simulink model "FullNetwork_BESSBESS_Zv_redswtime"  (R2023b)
settings: Solver=ode15s  StartTime=0.0  StopTime=140  RelTol=1e-3
PreLoadFcn:
  | Ts=50e-6;
model workspace (MAT data in the model file):
  Cf1 = 0.02
  Cf2 = 0.02
  Kffi1 = 0.9
  Kffi2 = 0.9
  Kffi3 = 0.9
  Kffv1 = 1
  Kffv2 = 1
  Kffv3 = 1
  Ki_cc1 = 5.9
  Ki_cc2 = 5.9
  Ki_cc3 = 5.9
  Ki_q1 = 0.0001
  Ki_q2 = 0.0001
  Ki_q3 = 0.0001
  Ki_vc1 = 150
  Ki_vc2 = 150
  Ki_vc3 = 150
  Kp_cc1 = 0.015
  Kp_cc2 = 0.015
  Kp_vc1 = 5
  Kp_vc2 = 5
  Kp_vc3 = 5
  Lf1 = 4.75e-06
  Lf2 = 4.75e-06
  Rf1 = 0.0005
  Rf2 = 0.0005
  Rf3 = 0.0005
  Rv1 = 0.0003169
  Rv2 = 0.0003169
  Snom1 = 100000000
  Snom2 = 100000000
  Vdc1 = 2000
  Vdc2 = 2000
  Vdc3 = 2000
  Xv1 = 0.0009509
  Xv2 = 0.0009509
  fnom1 = 50
  fnom2 = 50
  mp1 = 6.25e-08
  mp2 = 6.25e-08
  nq1 = 4.69166666667e-07
  nq2 = 4.69166666667e-07
  tau1 = 0.001
  tau2 = 0.001
  tau3 = 0.001
  vnom1 = 690
  vnom2 = 690
  vnom3 = 690
undefined symbols (not defined in the file or in its folder): Armidale, DiscIntNeverNeededParam, find_system, Gunnedah, Innerell, Ion, Lithium, Morree, Narrabri, Tamworth
libraries: spsThreePhaseBreakerLib x41, spsThreePhaseVIMeasurementLib x16, simulink_extras x16, spsThreePhaseSeriesRLCLoadLib x14, spsabctodq0Lib x12, spsThreePhaseTransformerTwoWindingsLib x11, slpidlib x8, spsLoadFlowBusLib x8, spsThreePhasePISectionLineLib x8, powerlib_extras x7, spsFirstOrderFilterLib x6, simulink x5
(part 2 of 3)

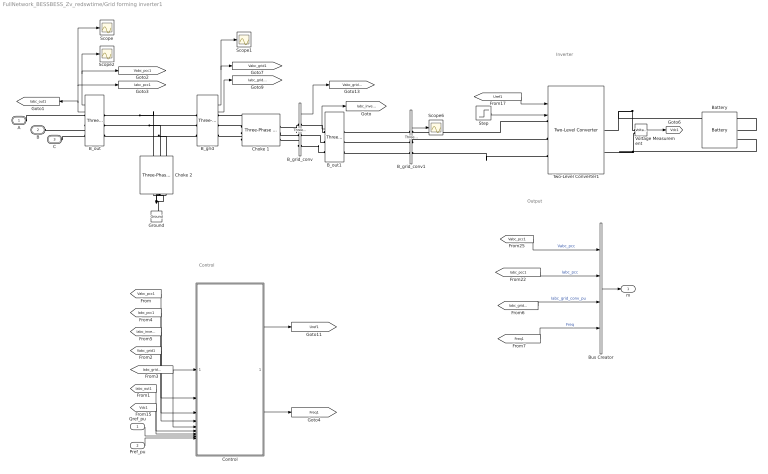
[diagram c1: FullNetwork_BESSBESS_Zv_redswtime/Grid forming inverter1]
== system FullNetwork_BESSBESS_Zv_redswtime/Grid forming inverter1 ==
  note: Control
  note: Inverter
  note: Output
  Qref_pu : Inport
  Pref_pu : Inport  Port=2
  B_grid : spsThreePhaseVIMeasurementLib/Three-Phase V-I Measurement  VoltageMeasurement=phase-to-ground  SetLabelV=off  LabelV=Vabc  Vpu=on  VpuLL=off  CurrentMeasurement=yes  SetLabelI=off  LabelI=Iabc  Ipu=on  Pbase=100e6  Vbase=690  OutputType=Complex  PhasorSimulation=off  PSBequivalent=0
  B_grid_conv : spsThreePhaseVIMeasurementLib/Three-Phase V-I Measurement  VoltageMeasurement=phase-to-ground  SetLabelV=off  LabelV=Vabc  Vpu=on  VpuLL=off  CurrentMeasurement=yes  SetLabelI=off  LabelI=Iabc  Ipu=off  Pbase=Pnom  Vbase=Vnom  OutputType=Complex  PhasorSimulation=off  PSBequivalent=0
  B_grid_conv1 : spsThreePhaseVIMeasurementLib/Three-Phase V-I Measurement  VoltageMeasurement=phase-to-ground  SetLabelV=off  LabelV=Vabc  Vpu=off  VpuLL=off  CurrentMeasurement=yes  SetLabelI=off  LabelI=Iabc  Ipu=off  Pbase=Pnom  Vbase=Vnom  OutputType=Complex  PhasorSimulation=off  PSBequivalent=0
  B_out : spsThreePhaseVIMeasurementLib/Three-Phase V-I Measurement  VoltageMeasurement=phase-to-ground  SetLabelV=off  LabelV=Vabc  Vpu=off  VpuLL=off  CurrentMeasurement=yes  SetLabelI=off  LabelI=Iabc  Ipu=off  Pbase=5e6  Vbase=690  OutputType=Complex  PhasorSimulation=off  PSBequivalent=0
  B_out1 : spsThreePhaseVIMeasurementLib/Three-Phase V-I Measurement  VoltageMeasurement=phase-to-ground  SetLabelV=off  LabelV=Vabc  Vpu=off  VpuLL=off  CurrentMeasurement=yes  SetLabelI=off  LabelI=Iabc  Ipu=off  Pbase=5e6  Vbase=690  OutputType=Complex  PhasorSimulation=off  PSBequivalent=0
  Battery : spsBatteryLib/Battery  BatType=Lithium-Ion  ShowTempParam=off  ThermalPreset=no  ShowAgeParam=off  NomV=2000  NomQ=200000  SOC=100  Batt_Tr=30  PresetModel=on  MaxQ=200000  MinV=1500  FullV=2327.9743  Dis_rate=86956.5217  R=0.0001  Normal_OP=180869.5652  expZone="[2160.7717       9826.087]"  current=[6.5 13 32.5]  Units=Time  Tci=20  NomT=20  T2=-30  MaxQ2=4.8  FullV2=7.1  Normal_OP2=5.655  expZone2="[6.58           1]"  Rca=0.6  ti=2000  Dp=0  Neq0=0  Tsim=1e6  Ta1=25  Qeol=5.4*0.9  Reol=0.013333*1.2  Char_age=[2.3478, 3]  Dis_age=[2.3478, 10]  N1=1500  N2=10500  N3=1000  N4=1400  Ta2=45  N5=950
  Bus Creator : BusCreator  Inputs=4
  Choke 1 : spsThreePhaseSeriesRLCBranchLib/Three-Phase Series RLC Branch  LConnTagsString=A|B|C  RConnTagsString=A|B|C  BranchType=RL  Resistance=Rf1  Inductance=Lf1  Capacitance=[]  Measurements=None
  Choke 2 : spsThreePhaseSeriesRLCBranchLib/Three-Phase Series RLC Branch  LConnTagsString=A|B|C  RConnTagsString=A|B|C  BranchType=C  Resistance=10e-3  Inductance=95e-6  Capacitance=Cf1  Measurements=None
  Control : Subsystem
  Ground : spsGroundLib/Ground  LConnTagsString=a
  Scope{,1..2,6} (4 alike) : Scope
  Step : Step  Time=2  SampleTime=0
  Two-Level Converter1 : spsTwoLevelConverterLib/Two-Level Converter  ModelType=Average model (No rectifier mode)  Ron=1e-3  Rs=1e6  Cs=inf  Vforward=[0,0]  Ron_Diode=1e-3  Rs_Diode=1e6  Cs_Diode=inf  Vf_Diode=1e-3  Rs_CurrentSource=inf  Ron_ACsource=1e-3
  Voltage Measurement : spsVoltageMeasurementLib/Voltage Measurement  PhasorSimulation=off  OutputType=Complex  PSBequivalent=0
  A : PMIOPort  Tag=PMCPort  Side=Left
  B : PMIOPort  Tag=PMCPort  Port=2  Side=Left
  C : PMIOPort  Tag=PMCPort  Port=3  Side=Left
  m : Outport  VectorParamsAs1DForOutWhenUnconnected=off
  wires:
  B_grid_conv/1 -> [Vabc_grid_conv1]
  B_grid/1 -> Scope1/1, [Vabc_grid1]
  B_grid/2 -> [Iabc_grid_conv1]
  [Vabc_grid1] -> Control/4(Vabc_grid)
  [Iabc_grid_conv1] -> Control/5(Iabc_grid_conv)
  [Vdc1] -> Control/7(Vdc)
  Qref_pu/1 -> Control/8(Qref)
  Control/1(Uref) -> [Uref1]
  [Uref1] -> Two-Level Converter1/1
  [Vabc_pcc1] -> Bus Creator/1  "Vabc_pcc"
  Bus Creator/1 -> m/1
  [Iabc_pcc1] -> Bus Creator/2  "Iabc_pcc"
  [Iabc_grid_conv1] -> Bus Creator/3  "Iabc_grid_conv_pu"
  [Iabc_out1] -> Control/6(Iabc_out)
  Pref_pu/1 -> Control/9(Pref_pu)
  Voltage Measurement/1 -> [Vdc1]
  B_out/1 -> [Vabc_pcc1], Scope2/1
  [Vabc_pcc1] -> Control/1(Vabc_pcc)
  [Iabc_pcc1] -> Control/2(Iabc_pcc)
  [Iabc_inverter1] -> Control/3(Iabc_inverter)
  B_out1/2 -> [Iabc_inverter1]
  B_grid_conv1/2 -> Scope6/1
  B_out/2 -> Scope/1, [Iabc_pcc1], [Iabc_out1]
  Control/2(Freq) -> [Freq1]
  [Freq1] -> Bus Creator/4  "Freq"
  Step/1 -> Two-Level Converter1/2
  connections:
  B_out/LConn1 -- Choke 2/LConn1 -- B_grid/LConn1
  B_out/LConn2 -- Choke 2/LConn2 -- B_grid/LConn2
  B_out/LConn3 -- Choke 2/LConn3 -- B_grid/LConn3
  Voltage Measurement/LConn2 -- Battery/LConn2 -- Two-Level Converter1/RConn2
  Voltage Measurement/LConn1 -- Battery/LConn1 -- Two-Level Converter1/RConn1
  C/RConn1 -- B_out/RConn3
  B_out/RConn2 -- B/RConn1
  A/RConn1 -- B_out/RConn1
  Two-Level Converter1/LConn1 -- B_grid_conv1/RConn1
  B_grid_conv1/RConn2 -- Two-Level Converter1/LConn2
  B_grid_conv1/RConn3 -- Two-Level Converter1/LConn3
  B_out1/LConn1 -- B_grid_conv1/LConn1
  B_out1/LConn3 -- B_grid_conv1/LConn3
  Choke 2/RConn2 -- Ground/LConn1 -- Choke 2/RConn1 -- Choke 2/RConn3
  B_grid_conv1/LConn2 -- B_out1/LConn2
  B_out1/RConn1 -- B_grid_conv/RConn1
  B_out1/RConn2 -- B_grid_conv/RConn2
  B_out1/RConn3 -- B_grid_conv/RConn3
  Choke 1/RConn2 -- B_grid_conv/LConn2
  B_grid_conv/LConn1 -- Choke 1/RConn1
  B_grid_conv/LConn3 -- Choke 1/RConn3
  Choke 1/LConn1 -- B_grid/RConn1
  Choke 1/LConn2 -- B_grid/RConn2
  Choke 1/LConn3 -- B_grid/RConn3

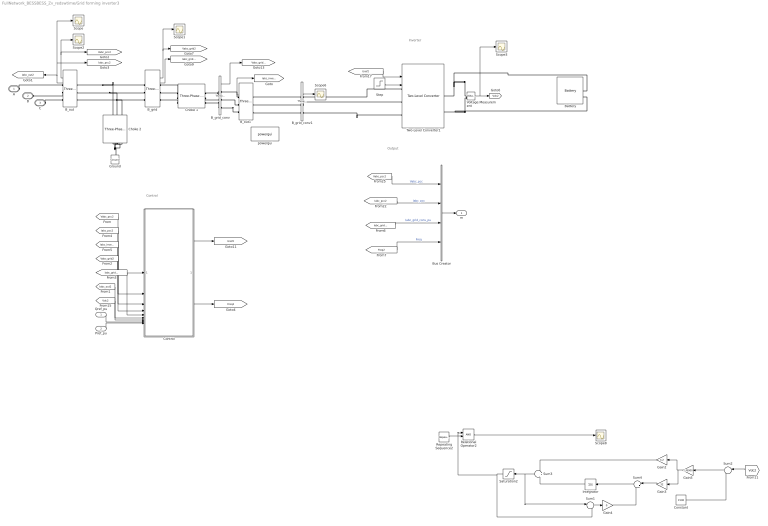
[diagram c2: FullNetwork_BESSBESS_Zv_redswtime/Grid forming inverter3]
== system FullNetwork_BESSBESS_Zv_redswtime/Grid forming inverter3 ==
  note: Control
  note: Inverter
  note: Output
  Qref_pu : Inport
  Pref_pu : Inport  Port=2
  B_grid : spsThreePhaseVIMeasurementLib/Three-Phase V-I Measurement  VoltageMeasurement=phase-to-ground  SetLabelV=off  LabelV=Vabc  Vpu=on  VpuLL=off  CurrentMeasurement=yes  SetLabelI=off  LabelI=Iabc  Ipu=on  Pbase=100e6  Vbase=690  OutputType=Complex  PhasorSimulation=off  PSBequivalent=0
  B_grid_conv : spsThreePhaseVIMeasurementLib/Three-Phase V-I Measurement  VoltageMeasurement=phase-to-ground  SetLabelV=off  LabelV=Vabc  Vpu=on  VpuLL=off  CurrentMeasurement=yes  SetLabelI=off  LabelI=Iabc  Ipu=off  Pbase=Pnom  Vbase=Vnom  OutputType=Complex  PhasorSimulation=off  PSBequivalent=0
  B_grid_conv1 : spsThreePhaseVIMeasurementLib/Three-Phase V-I Measurement  VoltageMeasurement=phase-to-ground  SetLabelV=off  LabelV=Vabc  Vpu=off  VpuLL=off  CurrentMeasurement=yes  SetLabelI=off  LabelI=Iabc  Ipu=off  Pbase=Pnom  Vbase=Vnom  OutputType=Complex  PhasorSimulation=off  PSBequivalent=0
  B_out : spsThreePhaseVIMeasurementLib/Three-Phase V-I Measurement  VoltageMeasurement=phase-to-ground  SetLabelV=off  LabelV=Vabc  Vpu=off  VpuLL=off  CurrentMeasurement=yes  SetLabelI=off  LabelI=Iabc  Ipu=off  Pbase=5e6  Vbase=690  OutputType=Complex  PhasorSimulation=off  PSBequivalent=0
  B_out1 : spsThreePhaseVIMeasurementLib/Three-Phase V-I Measurement  VoltageMeasurement=phase-to-ground  SetLabelV=off  LabelV=Vabc  Vpu=off  VpuLL=off  CurrentMeasurement=yes  SetLabelI=off  LabelI=Iabc  Ipu=off  Pbase=5e6  Vbase=690  OutputType=Complex  PhasorSimulation=off  PSBequivalent=0
  Battery : spsBatteryLib/Battery  BatType=Lithium-Ion  ShowTempParam=off  ThermalPreset=no  ShowAgeParam=off  NomV=2000  NomQ=200000  SOC=100  Batt_Tr=30  PresetModel=on  MaxQ=200000  MinV=1500  FullV=2327.9743  Dis_rate=86956.5217  R=0.0001  Normal_OP=180869.5652  expZone="[2160.7717       9826.087]"  current=[6.5 13 32.5]  Units=Time  Tci=20  NomT=20  T2=-30  MaxQ2=4.8  FullV2=7.1  Normal_OP2=5.655  expZone2="[6.58           1]"  Rca=0.6  ti=2000  Dp=0  Neq0=0  Tsim=1e6  Ta1=25  Qeol=5.4*0.9  Reol=0.013333*1.2  Char_age=[2.3478, 3]  Dis_age=[2.3478, 10]  N1=1500  N2=10500  N3=1000  N4=1400  Ta2=45  N5=950
  Bus Creator : BusCreator  Inputs=4
  Choke 1 : spsThreePhaseSeriesRLCBranchLib/Three-Phase Series RLC Branch  LConnTagsString=A|B|C  RConnTagsString=A|B|C  BranchType=RL  Resistance=Rf2  Inductance=Lf2  Capacitance=[]  Measurements=None
  Choke 2 : spsThreePhaseSeriesRLCBranchLib/Three-Phase Series RLC Branch  LConnTagsString=A|B|C  RConnTagsString=A|B|C  BranchType=C  Resistance=10e-3  Inductance=95e-6  Capacitance=Cf2  Measurements=None
  Constant : Constant  Value=1500
  Control : Subsystem
  Gain2 : Gain  Gain=3.2
  Gain3 : Gain  Gain=32
  Gain4 : Gain  Gain=0
  Gain5 : Gain  Gain=-1/8000
  Ground : spsGroundLib/Ground  LConnTagsString=a
  Integrator : Integrator
  Relational Operator2 : RelationalOperator  OutDataTypeStr=boolean
  Repeating Sequence2 : simulink/Sources/Repeating Sequence  rep_seq_t=[0 1000e-6 2000e-6]  rep_seq_y=[0 1 0]
  Saturation2 : Saturate  UpperLimit=0.95  LowerLimit=0
  Scope{,1..3,6,8} (6 alike) : Scope
  Step : Step  Time=0  SampleTime=0
  Sum1 : Sum  Inputs=|-+
  Sum2 : Sum  Inputs=|-+
  Sum3 : Sum
  Sum4 : Sum  Inputs=|++
  Two-Level Converter1 : spsTwoLevelConverterLib/Two-Level Converter  ModelType=Average model (No rectifier mode)  Ron=1e-3  Rs=1e6  Cs=inf  Vforward=[0,0]  Ron_Diode=1e-3  Rs_Diode=1e6  Cs_Diode=inf  Vf_Diode=1e-3  Rs_CurrentSource=inf  Ron_ACsource=1e-3
  Voltage Measurement : spsVoltageMeasurementLib/Voltage Measurement  PhasorSimulation=off  OutputType=Complex  PSBequivalent=0
  powergui : spspowerguiLib/powergui  Priority=1  SimulationMode=Discrete  SampleTime=50e-6  frequency=60  Iterations=50  frequencyindice=60  Pbase=100e6  ErrMax=1e-4  UnitsV=kV  UnitsW=MW  buscounter=0  FunctionMessages=off  echomessages=off  EnableUseOfTLC=off  CurrentSourceSwitches=off  DisableSnubberDevices=off  DisableRonSwitches=off  DisableVfSwitches=off  DisplayEquations=off  AutomaticDiscreteSolvers=off  SolverType=Tustin/Backward Euler (TBE)  Interpol=off  ExternalGateDelay=off  methode=off  Ts=100  x0status=blocks  SPID=on  SwTol=0  HookPort=off  NonlinearTolerance=1e-4  nMaxIteration=100  ContinueOnMaxIteration=off  RestoreLinks=warning  ResistiveCurrentMeasurement=off  Frange=[0:2:500]  Ylog=off  Xlog=on  ShowGrid=off  save=off  variable=ZData  structure=0  ZoomFFT=off  StartTime=0.0  cycles=1  DisplayStyle=1  fundamental=60  FreqAxis=off  MaxFrequency=1000  frequencyindicesteady=1  RmsSteady=1  display=off
  A : PMIOPort  Tag=PMCPort  Side=Left
  B : PMIOPort  Tag=PMCPort  Port=2  Side=Left
  C : PMIOPort  Tag=PMCPort  Port=3  Side=Left
  m : Outport  VectorParamsAs1DForOutWhenUnconnected=off
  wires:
  B_grid_conv/1 -> [Vabc_grid_conv2]
  B_grid/1 -> Scope1/1, [Vabc_grid2]
  B_grid/2 -> [Iabc_grid_conv2]
  [Vabc_grid2] -> Control/4(Vabc_grid)
  [Iabc_grid_conv2] -> Control/5(Iabc_grid_conv)
  [Vdc2] -> Control/7(Vdc)
  Qref_pu/1 -> Control/8(Qref)
  Control/1(Uref) -> [Uref2]
  [Uref2] -> Two-Level Converter1/1
  [Vabc_pcc2] -> Bus Creator/1  "Vabc_pcc"
  Bus Creator/1 -> m/1
  [Iabc_pcc2] -> Bus Creator/2  "Iabc_pcc"
  [Iabc_grid_conv2] -> Bus Creator/3  "Iabc_grid_conv_pu"
  [Iabc_out2] -> Control/6(Iabc_out)
  Pref_pu/1 -> Control/9(Pref_pu)
  Voltage Measurement/1 -> Scope3/1, [Vdc2]
  B_out/1 -> [Vabc_pcc2], Scope2/1
  [Vabc_pcc2] -> Control/1(Vabc_pcc)
  [Iabc_pcc2] -> Control/2(Iabc_pcc)
  [Iabc_inverter2] -> Control/3(Iabc_inverter)
  B_out1/2 -> [Iabc_inverter2]
  B_grid_conv1/2 -> Scope6/1
  B_out/2 -> Scope/1, [Iabc_pcc2], [Iabc_out2]
  Control/2(Freq) -> [Freq2]
  [Freq2] -> Bus Creator/4  "Freq"
  Step/1 -> Two-Level Converter1/2
  Constant/1 -> Sum2/2
  Sum2/1 -> Gain5/1
  Integrator/1 -> Sum3/2
  [Vdc2] -> Sum2/1
  Gain5/1 -> Gain3/1, Gain2/1
  Sum3/1 -> Sum1/1, Saturation2/1
  Sum1/1 -> Gain4/1
  Saturation2/1 -> Relational Operator2/1, Sum1/2
  Gain3/1 -> Sum4/1
  Relational Operator2/1 -> Scope8/1
  Sum4/1 -> Integrator/1
  Gain4/1 -> Sum4/2
  Repeating Sequence2/1 -> Relational Operator2/2
  Gain2/1 -> Sum3/1
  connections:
  B_out/LConn1 -- Choke 2/LConn1 -- B_grid/LConn1
  B_out/LConn2 -- Choke 2/LConn2 -- B_grid/LConn2
  B_out/LConn3 -- Choke 2/LConn3 -- B_grid/LConn3
  Voltage Measurement/LConn2 -- Battery/LConn2 -- Two-Level Converter1/RConn2
  C/RConn1 -- B_out/RConn3
  B_out/RConn2 -- B/RConn1
  A/RConn1 -- B_out/RConn1
  Two-Level Converter1/LConn1 -- B_grid_conv1/RConn1
  B_grid_conv1/RConn2 -- Two-Level Converter1/LConn2
  B_grid_conv1/RConn3 -- Two-Level Converter1/LConn3
  B_out1/LConn1 -- B_grid_conv1/LConn1
  B_out1/LConn3 -- B_grid_conv1/LConn3
  Choke 2/RConn2 -- Ground/LConn1 -- Choke 2/RConn1 -- Choke 2/RConn3
  B_grid_conv1/LConn2 -- B_out1/LConn2
  B_out1/RConn1 -- B_grid_conv/RConn1
  B_out1/RConn2 -- B_grid_conv/RConn2
  B_out1/RConn3 -- B_grid_conv/RConn3
  Choke 1/RConn2 -- B_grid_conv/LConn2
  B_grid_conv/LConn1 -- Choke 1/RConn1
  B_grid_conv/LConn3 -- Choke 1/RConn3
  Choke 1/LConn1 -- B_grid/RConn1
  Choke 1/LConn2 -- B_grid/RConn2
  Choke 1/LConn3 -- B_grid/RConn3
  Voltage Measurement/LConn1 -- Battery/LConn1 -- Two-Level Converter1/RConn1

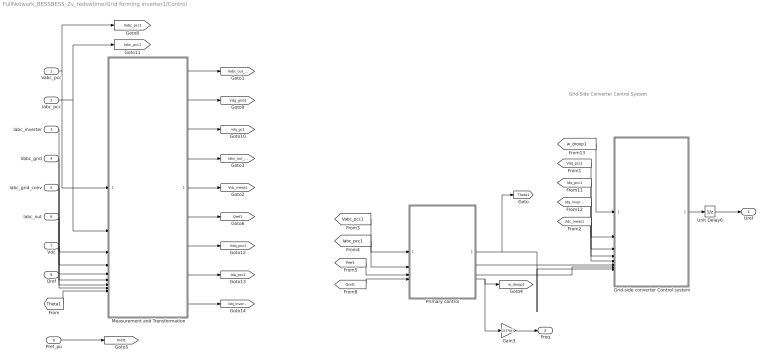
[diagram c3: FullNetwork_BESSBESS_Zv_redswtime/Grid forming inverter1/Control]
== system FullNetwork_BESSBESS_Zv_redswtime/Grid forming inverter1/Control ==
  note: Grid-Side Converter Control System
  Vabc_pcc : Inport
  Iabc_pcc : Inport  Port=2
  Iabc_inverter : Inport  Port=3
  Vabc_grid : Inport  Port=4
  Iabc_grid_conv : Inport  Port=5
  Iabc_out : Inport  Port=6
  Vdc : Inport  Port=7
  Qref : Inport  Port=8
  Pref_pu : Inport  Port=9
  Gain3 : Gain  Gain=1/(2*pi)
  Grid-side converter Control system : Subsystem
  Measurement and Transformation : Subsystem
  Primary control : Subsystem  Variant=on  VariantControl=Choice
  Unit Delay6 : UnitDelay  SampleTime=Ts  HasFrameUpgradeWarning=on
  Uref : Outport  VectorParamsAs1DForOutWhenUnconnected=off
  Freq : Outport  Port=2  VectorParamsAs1DForOutWhenUnconnected=off
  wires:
  [Vdq_pcc1] -> Grid-side converter Control system/2(Vdq_pcc)
  [Vdc_meas1] -> Grid-side converter Control system/5(Vdc)
  Grid-side converter Control system/1(Uctrl_inverter) -> Unit Delay6/1
  Unit Delay6/1 -> Uref/1
  Vabc_grid/1 -> Measurement and Transformation/4(Vabc_grid)
  Iabc_grid_conv/1 -> Measurement and Transformation/5(Iabc_gc)
  Vdc/1 -> Measurement and Transformation/7(Vdc)
  Qref/1 -> Measurement and Transformation/8(Qref)
  Measurement and Transformation/2(Vdq_grid) -> [Vdq_grid1]
  Measurement and Transformation/3(Idq_gc) -> [Idq_gc1]
  Measurement and Transformation/5(Vdc_meas) -> [Vdc_meas1]
  Measurement and Transformation/6("Qref ") -> [Qref1]
  Iabc_out/1 -> Measurement and Transformation/6(Iabc_out)
  [Theta1] -> Measurement and Transformation/9(Theta)
  Measurement and Transformation/4(I_abc_out) -> [Iabc_out_pu1]
  Measurement and Transformation/1(V_abc_grid) -> [Vabc_out_pu1]
  Pref_pu/1 -> [Pref1]
  Vabc_pcc/1 -> [Vabc_pcc1], Measurement and Transformation/1(Vabc_pcc)
  Iabc_pcc/1 -> [Iabc_pcc1], Measurement and Transformation/2(Iabc_pcc)
  Iabc_inverter/1 -> Measurement and Transformation/3(Iabc_inverter)
  [Idq_pcc1] -> Grid-side converter Control system/3(Idq_pcc)
  [Idq_inverter1] -> Grid-side converter Control system/4(Idq_inverter)
  Measurement and Transformation/7(Vdq_pcc) -> [Vdq_pcc1]
  Measurement and Transformation/8(Idq_pcc) -> [Idq_pcc1]
  Measurement and Transformation/9(Idq_inverter) -> [Idq_inverter1]
  [w_droop1] -> Grid-side converter Control system/1(w)
  [Vabc_pcc1] -> Primary control/1(Vabc_pu)
  [Iabc_pcc1] -> Primary control/2(Iabc_pu)
  [Pref1] -> Primary control/3(Pref_pu)
  [Qref1] -> Primary control/4(Qref_pu)
  Primary control/1(Theta) -> Grid-side converter Control system/8(Theta_PLL), [Theta1]
  Primary control/2(Vd_ref) -> Grid-side converter Control system/6(Vd_ref)
  Primary control/3(Vq_ref) -> Grid-side converter Control system/7(Vq_ref)
  Primary control/4(w_droop) -> Gain3/1, [w_droop1]
  Gain3/1 -> Freq/1

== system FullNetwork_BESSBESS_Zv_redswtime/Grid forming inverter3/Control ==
  note: Grid-Side Converter Control System
  Vabc_pcc : Inport
  Iabc_pcc : Inport  Port=2
  Iabc_inverter : Inport  Port=3
  Vabc_grid : Inport  Port=4
  Iabc_grid_conv : Inport  Port=5
  Iabc_out : Inport  Port=6
  Vdc : Inport  Port=7
  Qref : Inport  Port=8
  Pref_pu : Inport  Port=9
  Gain3 : Gain  Gain=1/(2*pi)
  Grid-side converter Control system : Subsystem
  Measurement and Transformation : Subsystem
  Primary control : Subsystem  Variant=on  VariantControl=Choice
  Unit Delay6 : UnitDelay  SampleTime=Ts  HasFrameUpgradeWarning=on
  Uref : Outport  VectorParamsAs1DForOutWhenUnconnected=off
  Freq : Outport  Port=2  VectorParamsAs1DForOutWhenUnconnected=off
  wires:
  [Vdq_pcc2] -> Grid-side converter Control system/2(Vdq_pcc)
  [Vdc_meas2] -> Grid-side converter Control system/5(Vdc)
  Grid-side converter Control system/1(Uctrl_inverter) -> Unit Delay6/1
  Unit Delay6/1 -> Uref/1
  Vabc_grid/1 -> Measurement and Transformation/4(Vabc_grid)
  Iabc_grid_conv/1 -> Measurement and Transformation/5(Iabc_gc)
  Vdc/1 -> Measurement and Transformation/7(Vdc)
  Qref/1 -> Measurement and Transformation/8(Qref)
  Measurement and Transformation/2(Vdq_grid) -> [Vdq_grid2]
  Measurement and Transformation/3(Idq_gc) -> [Idq_gc2]
  Measurement and Transformation/5(Vdc_meas) -> [Vdc_meas2]
  Measurement and Transformation/6("Qref ") -> [Qref2]
  Iabc_out/1 -> Measurement and Transformation/6(Iabc_out)
  [Theta2] -> Measurement and Transformation/9(Theta)
  Measurement and Transformation/4(I_abc_out) -> [Iabc_out_pu2]
  Measurement and Transformation/1(V_abc_grid) -> [Vabc_out_pu2]
  Pref_pu/1 -> [Pref1]
  Vabc_pcc/1 -> [Vabc_pcc2], Measurement and Transformation/1(Vabc_pcc)
  Iabc_pcc/1 -> [Iabc_pcc2], Measurement and Transformation/2(Iabc_pcc)
  Iabc_inverter/1 -> Measurement and Transformation/3(Iabc_inverter)
  [Idq_pcc2] -> Grid-side converter Control system/3(Idq_pcc)
  [Idq_inverter2] -> Grid-side converter Control system/4(Idq_inverter)
  Measurement and Transformation/7(Vdq_pcc) -> [Vdq_pcc2]
  Measurement and Transformation/8(Idq_pcc) -> [Idq_pcc2]
  Measurement and Transformation/9(Idq_inverter) -> [Idq_inverter2]
  [w_droop2] -> Grid-side converter Control system/1(w)
  [Vabc_pcc2] -> Primary control/1(Vabc_pu)
  [Iabc_pcc2] -> Primary control/2(Iabc_pu)
  [Pref2] -> Primary control/3(Pref_pu)
  [Qref2] -> Primary control/4(Qref_pu)
  Primary control/1(Theta) -> Grid-side converter Control system/8(Theta_PLL), [Theta2]
  Primary control/2(Vd_ref) -> Grid-side converter Control system/6(Vd_ref)
  Primary control/3(Vq_ref) -> Grid-side converter Control system/7(Vq_ref)
  Primary control/4(w_droop) -> Gain3/1, [w_droop2]
  Gain3/1 -> Freq/1

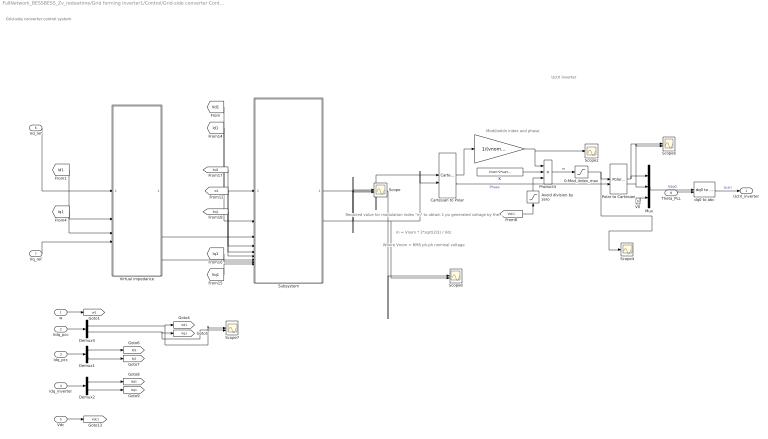
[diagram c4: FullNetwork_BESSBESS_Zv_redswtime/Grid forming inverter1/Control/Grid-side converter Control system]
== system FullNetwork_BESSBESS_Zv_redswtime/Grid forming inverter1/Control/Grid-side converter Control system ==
  note: Modulation index and phase
  note: Where Vnom = RMS ph-ph nominal voltage
  note: m = Vnom * 2*sqrt(2/3) / Vdc
  note: Required value for modulation index "m" to obtain 1 pu generated voltage by the converter:
  note: Grid-side converter control system
  note: Uctrl inverter
  w : Inport
  Vdq_pcc : Inport  Port=2
  Idq_pcc : Inport  Port=3
  Idq_inverter : Inport  Port=4
  Vdc : Inport  Port=5
  Vd_ref : Inport  Port=6
  Vq_ref : Inport  Port=7
  Theta_PLL : Inport  Port=8
  0-Mod_index_max : Saturate  UpperLimit=Mod_index_max*0+1.4  LowerLimit=0
  Avoid division by zero : Saturate  UpperLimit=1e6  LowerLimit=1e-6
  Cartesian to Polar : simulink_extras/Transformations/Cartesian to Polar
  Demux1 : Demux  Outputs=2
  Demux2 : Demux  Outputs=2
  Demux4 : Demux  Outputs=2
  Gain8 : Gain  Gain=1/(vnom1*sqrt(2/3))
  K : Constant  Value=Vnom*2*sqrt(2/3)
  Mux : Mux  Inputs=3
  Polar to Cartesian : simulink_extras/Transformations/Polar to Cartesian
  Product4 : Product  Inputs=**/  InputSameDT=on  SaturateOnIntegerOverflow=on
  Scope{,6..8} (4 alike) : Scope  NumInputPorts=2
  Scope2 : Scope
  Scope4 : Scope
  Subsystem : Subsystem  Variant=on  VariantControl=Choice
  V0 : Constant  Value=0
  Virtual impedance : Subsystem  Variant=on  VariantControl=Choice
  dq0 to abc : spsdq0toabcLib/dq0 to abc  Alignment=90 degrees behind phase A axis
  Uctrl_inverter : Outport  VectorParamsAs1DForOutWhenUnconnected=off
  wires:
  0-Mod_index_max/1 -> Polar to Cartesian/1, Scope4/1
  Cartesian to Polar/2 -> Polar to Cartesian/2  "Phase"
  [Vdc1] -> Avoid division by zero/1
  Cartesian to Polar/1 -> Gain8/1
  Avoid division by zero/1 -> Product4/3
  K/1 -> Product4/2
  Product4/1 -> 0-Mod_index_max/1  "m"
  Demux4/2 -> Scope7/2, [Vq1]
  Demux4/1 -> Scope7/1, [Vd1]
  w/1 -> [w1]
  Vdq_pcc/1 -> Demux4/1
  Vdc/1 -> [Vdc1]
  Idq_pcc/1 -> Demux1/1
  Demux1/1 -> [Id1]
  Demux1/2 -> [Iq1]
  Demux2/2 -> [Itq1]
  Demux2/1 -> [Itd1]
  Idq_inverter/1 -> Demux2/1
  Polar to Cartesian/1 -> Mux/1, Scope6/1
  Theta_PLL/1 -> dq0 to abc/2
  V0/1 -> Mux/3
  Polar to Cartesian/2 -> Mux/2, Scope6/2
  Mux/1 -> dq0 to abc/1  "Vdq0"
  dq0 to abc/1 -> Uctrl_inverter/1  "Uctrl"
  Gain8/1 -> Product4/1, Scope2/1
  Vd_ref/1 -> Virtual impedance/1(Vd_ref)
  [Id1] -> Virtual impedance/2(Id)
  [Iq1] -> Virtual impedance/3(Iq)
  Vq_ref/1 -> Virtual impedance/4(Vq_ref)
  Subsystem/1(Vd inverter) -> Scope/1, Scope8/1, Cartesian to Polar/1
  Subsystem/2(Vq inverter) -> Scope/2, Cartesian to Polar/2, Scope8/2
  [Vd1] -> Subsystem/1(Vd)
  [Id1] -> Subsystem/2(Id)
  [Vq1] -> Subsystem/9(Vq)
  Virtual impedance/1(Vd_ref*) -> Subsystem/3(Vd_ref)
  [Iq1] -> Subsystem/8(Iq)
  [Itd1] -> Subsystem/4(Itd)
  Virtual impedance/2(Vq_ref*) -> Subsystem/7(Vq_ref)
  [w1] -> Subsystem/5(w)
  [Itq1] -> Subsystem/6(Itq)

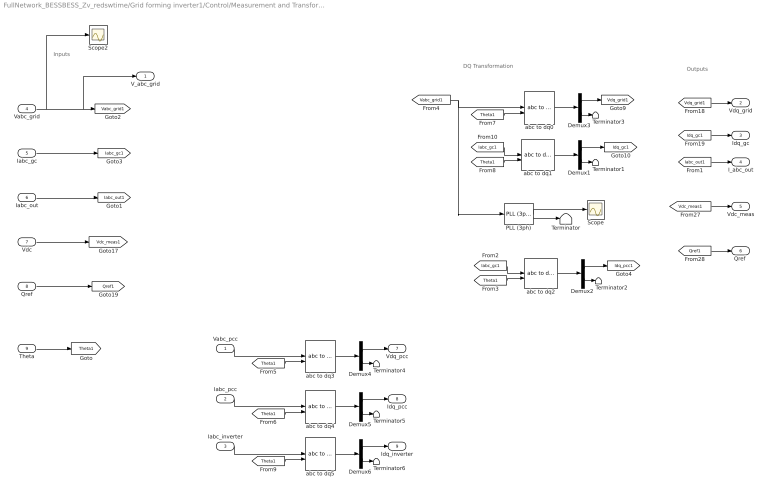
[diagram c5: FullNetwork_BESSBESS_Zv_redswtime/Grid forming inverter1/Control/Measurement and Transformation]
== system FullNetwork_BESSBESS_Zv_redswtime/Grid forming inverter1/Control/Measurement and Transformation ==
  note: Inputs
  note: DQ Transformation
  note: Outputs
  Vabc_pcc : Inport
  Iabc_pcc : Inport  Port=2
  Iabc_inverter : Inport  Port=3
  Vabc_grid : Inport  Port=4
  Iabc_gc : Inport  Port=5
  Iabc_out : Inport  Port=6
  Vdc : Inport  Port=7
  Qref : Inport  Port=8
  Theta : Inport  Port=9
  Demux{1..6} (6 alike) : Demux  Outputs=[2 1]
  PLL (3ph) : spsPLL3phLib/PLL (3ph)  Fmin=35  Par_Init=[0, 50]  ParK=[180, 3200, 0]  TcD=1e-4  MaxRateChangeFreq=12  FilterCutOffFreq=25  Ts=Ts  AGC=on
  Scope : Scope
  Scope2 : Scope
  Terminator{,1..6} (7 alike) : Terminator
  abc to dq{0..5} (6 alike) : spsabctodq0Lib/abc to dq0  Alignment=90 degrees behind phase A axis
  V_abc_grid : Outport  VectorParamsAs1DForOutWhenUnconnected=off
  Vdq_grid : Outport  Port=2  VectorParamsAs1DForOutWhenUnconnected=off
  Idq_gc : Outport  Port=3  VectorParamsAs1DForOutWhenUnconnected=off
  I_abc_out : Outport  Port=4  VectorParamsAs1DForOutWhenUnconnected=off
  Vdc_meas : Outport  Port=5  VectorParamsAs1DForOutWhenUnconnected=off
  "Qref " : Outport  Port=6  VectorParamsAs1DForOutWhenUnconnected=off
  Vdq_pcc : Outport  Port=7  VectorParamsAs1DForOutWhenUnconnected=off
  Idq_pcc : Outport  Port=8  VectorParamsAs1DForOutWhenUnconnected=off
  Idq_inverter : Outport  Port=9  VectorParamsAs1DForOutWhenUnconnected=off
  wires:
  Qref/1 -> [Qref1]
  Vdc/1 -> [Vdc_meas1]
  Iabc_gc/1 -> [Iabc_gc1]
  Vabc_grid/1 -> V_abc_grid/1, [Vabc_grid1], Scope2/1
  [Qref1] -> "Qref "/1
  [Vdc_meas1] -> Vdc_meas/1
  [Idq_gc1] -> Idq_gc/1
  [Vdq_grid1] -> Vdq_grid/1
  Demux1/1 -> [Idq_gc1]
  [Iabc_gc1] -> abc to dq1/1
  [Theta1] -> abc to dq1/2
  [Vabc_grid1] -> PLL (3ph)/1, abc to dq0/1
  abc to dq0/1 -> Demux3/1
  abc to dq1/1 -> Demux1/1
  Demux3/2 -> Terminator3/1
  Demux3/1 -> [Vdq_grid1]
  Demux1/2 -> Terminator1/1
  Theta/1 -> [Theta1]
  Iabc_out/1 -> [Iabc_out1]
  [Iabc_out1] -> I_abc_out/1
  PLL (3ph)/2 -> Terminator/1
  PLL (3ph)/1 -> Scope/1
  [Theta1] -> abc to dq0/2
  Demux2/1 -> [Idq_pcc1]
  abc to dq2/1 -> Demux2/1
  [Theta1] -> abc to dq2/2
  Demux2/2 -> Terminator2/1
  [Iabc_gc1] -> abc to dq2/1
  abc to dq3/1 -> Demux4/1
  [Theta1] -> abc to dq3/2
  Demux4/2 -> Terminator4/1
  Demux4/1 -> Vdq_pcc/1
  [Theta1] -> abc to dq4/2
  Demux5/2 -> Terminator5/1
  Demux5/1 -> Idq_pcc/1
  abc to dq4/1 -> Demux5/1
  Demux6/2 -> Terminator6/1
  abc to dq5/1 -> Demux6/1
  Demux6/1 -> Idq_inverter/1
  [Theta1] -> abc to dq5/2
  Vabc_pcc/1 -> abc to dq3/1
  Iabc_pcc/1 -> abc to dq4/1
  Iabc_inverter/1 -> abc to dq5/1

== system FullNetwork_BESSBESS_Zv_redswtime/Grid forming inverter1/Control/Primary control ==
  Vabc_pu : Inport
  Iabc_pu : Inport  Port=2
  Pref_pu : Inport  Port=3
  Qref_pu : Inport  Port=4
  Droop : Subsystem  VariantControl=ControlType == 1
  Virtual synchronous machine : Subsystem  VariantControl=ControlType == 2
  Theta : Outport
  Vd_ref : Outport  Port=2
  Vq_ref : Outport  Port=3
  w_droop : Outport  Port=4

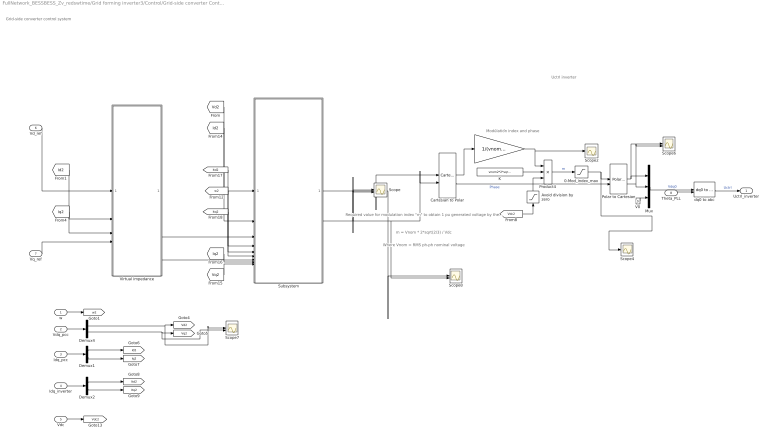
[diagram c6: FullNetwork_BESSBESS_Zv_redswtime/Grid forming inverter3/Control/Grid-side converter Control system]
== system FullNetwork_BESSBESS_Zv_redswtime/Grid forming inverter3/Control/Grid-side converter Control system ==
  note: Modulation index and phase
  note: Where Vnom = RMS ph-ph nominal voltage
  note: m = Vnom * 2*sqrt(2/3) / Vdc
  note: Required value for modulation index "m" to obtain 1 pu generated voltage by the converter:
  note: Grid-side converter control system
  note: Uctrl inverter
  w : Inport
  Vdq_pcc : Inport  Port=2
  Idq_pcc : Inport  Port=3
  Idq_inverter : Inport  Port=4
  Vdc : Inport  Port=5
  Vd_ref : Inport  Port=6
  Vq_ref : Inport  Port=7
  Theta_PLL : Inport  Port=8
  0-Mod_index_max : Saturate  UpperLimit=Mod_index_max*0+1.4  LowerLimit=0
  Avoid division by zero : Saturate  UpperLimit=1e6  LowerLimit=1e-6
  Cartesian to Polar : simulink_extras/Transformations/Cartesian to Polar
  Demux1 : Demux  Outputs=2
  Demux2 : Demux  Outputs=2
  Demux4 : Demux  Outputs=2
  Gain8 : Gain  Gain=1/(vnom2*sqrt(2/3))
  K : Constant  Value=vnom2*2*sqrt(2/3)
  Mux : Mux  Inputs=3
  Polar to Cartesian : simulink_extras/Transformations/Polar to Cartesian
  Product4 : Product  Inputs=**/  InputSameDT=on  SaturateOnIntegerOverflow=on
  Scope{,6..8} (4 alike) : Scope  NumInputPorts=2
  Scope2 : Scope
  Scope4 : Scope
  Subsystem : Subsystem  Variant=on  VariantControl=Choice
  V0 : Constant  Value=0
  Virtual impedance : Subsystem  Variant=on  VariantControl=Choice
  dq0 to abc : spsdq0toabcLib/dq0 to abc  Alignment=90 degrees behind phase A axis
  Uctrl_inverter : Outport  VectorParamsAs1DForOutWhenUnconnected=off
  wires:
  0-Mod_index_max/1 -> Polar to Cartesian/1, Scope4/1
  Cartesian to Polar/2 -> Polar to Cartesian/2  "Phase"
  [Vdc2] -> Avoid division by zero/1
  Cartesian to Polar/1 -> Gain8/1
  Avoid division by zero/1 -> Product4/3
  K/1 -> Product4/2
  Product4/1 -> 0-Mod_index_max/1  "m"
  Demux4/2 -> Scope7/2, [Vq2]
  Demux4/1 -> Scope7/1, [Vd2]
  w/1 -> [w2]
  Vdq_pcc/1 -> Demux4/1
  Vdc/1 -> [Vdc2]
  Idq_pcc/1 -> Demux1/1
  Demux1/1 -> [Id2]
  Demux1/2 -> [Iq2]
  Demux2/2 -> [Itq2]
  Demux2/1 -> [Itd2]
  Idq_inverter/1 -> Demux2/1
  Polar to Cartesian/1 -> Mux/1, Scope6/1
  Theta_PLL/1 -> dq0 to abc/2
  V0/1 -> Mux/3
  Polar to Cartesian/2 -> Mux/2, Scope6/2
  Mux/1 -> dq0 to abc/1  "Vdq0"
  dq0 to abc/1 -> Uctrl_inverter/1  "Uctrl"
  Gain8/1 -> Product4/1, Scope2/1
  Vd_ref/1 -> Virtual impedance/1(Vd_ref)
  [Id2] -> Virtual impedance/2(Id)
  [Iq2] -> Virtual impedance/3(Iq)
  Vq_ref/1 -> Virtual impedance/4(Vq_ref)
  Subsystem/1(Vd inverter) -> Scope/1, Scope8/1, Cartesian to Polar/1
  Subsystem/2(Vq inverter) -> Scope/2, Cartesian to Polar/2, Scope8/2
  [Vd2] -> Subsystem/1(Vd)
  [Id2] -> Subsystem/2(Id)
  [Vq2] -> Subsystem/9(Vq)
  Virtual impedance/1(Vd_ref*) -> Subsystem/3(Vd_ref)
  [Iq2] -> Subsystem/8(Iq)
  [Itd2] -> Subsystem/4(Itd)
  Virtual impedance/2(Vq_ref*) -> Subsystem/7(Vq_ref)
  [w2] -> Subsystem/5(w)
  [Itq2] -> Subsystem/6(Itq)

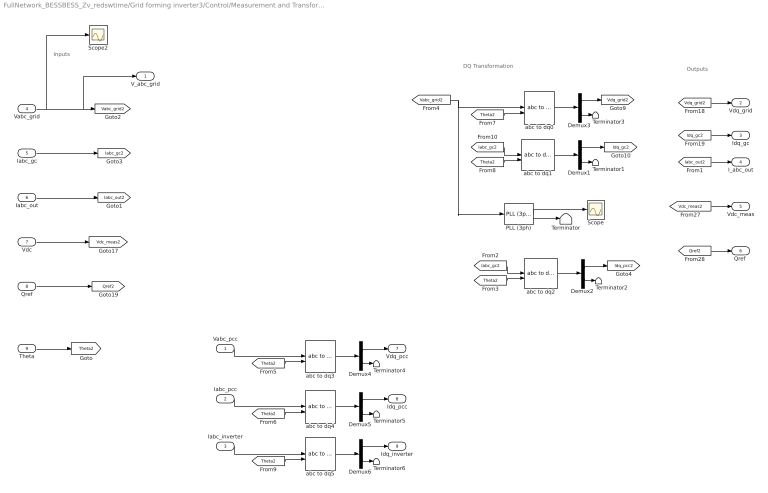
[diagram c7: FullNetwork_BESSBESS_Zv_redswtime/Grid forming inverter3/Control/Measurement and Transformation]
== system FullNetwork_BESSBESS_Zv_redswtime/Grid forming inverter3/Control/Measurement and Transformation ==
  note: Inputs
  note: DQ Transformation
  note: Outputs
  Vabc_pcc : Inport
  Iabc_pcc : Inport  Port=2
  Iabc_inverter : Inport  Port=3
  Vabc_grid : Inport  Port=4
  Iabc_gc : Inport  Port=5
  Iabc_out : Inport  Port=6
  Vdc : Inport  Port=7
  Qref : Inport  Port=8
  Theta : Inport  Port=9
  Demux{1..6} (6 alike) : Demux  Outputs=[2 1]
  PLL (3ph) : spsPLL3phLib/PLL (3ph)  Fmin=35  Par_Init=[0, 50]  ParK=[180, 3200, 0]  TcD=1e-4  MaxRateChangeFreq=12  FilterCutOffFreq=25  Ts=Ts  AGC=on
  Scope : Scope
  Scope2 : Scope
  Terminator{,1..6} (7 alike) : Terminator
  abc to dq{0..5} (6 alike) : spsabctodq0Lib/abc to dq0  Alignment=90 degrees behind phase A axis
  V_abc_grid : Outport  VectorParamsAs1DForOutWhenUnconnected=off
  Vdq_grid : Outport  Port=2  VectorParamsAs1DForOutWhenUnconnected=off
  Idq_gc : Outport  Port=3  VectorParamsAs1DForOutWhenUnconnected=off
  I_abc_out : Outport  Port=4  VectorParamsAs1DForOutWhenUnconnected=off
  Vdc_meas : Outport  Port=5  VectorParamsAs1DForOutWhenUnconnected=off
  "Qref " : Outport  Port=6  VectorParamsAs1DForOutWhenUnconnected=off
  Vdq_pcc : Outport  Port=7  VectorParamsAs1DForOutWhenUnconnected=off
  Idq_pcc : Outport  Port=8  VectorParamsAs1DForOutWhenUnconnected=off
  Idq_inverter : Outport  Port=9  VectorParamsAs1DForOutWhenUnconnected=off
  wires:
  Qref/1 -> [Qref2]
  Vdc/1 -> [Vdc_meas2]
  Iabc_gc/1 -> [Iabc_gc2]
  Vabc_grid/1 -> V_abc_grid/1, [Vabc_grid2], Scope2/1
  [Qref2] -> "Qref "/1
  [Vdc_meas2] -> Vdc_meas/1
  [Idq_gc2] -> Idq_gc/1
  [Vdq_grid2] -> Vdq_grid/1
  Demux1/1 -> [Idq_gc2]
  [Iabc_gc2] -> abc to dq1/1
  [Theta2] -> abc to dq1/2
  [Vabc_grid2] -> PLL (3ph)/1, abc to dq0/1
  abc to dq0/1 -> Demux3/1
  abc to dq1/1 -> Demux1/1
  Demux3/2 -> Terminator3/1
  Demux3/1 -> [Vdq_grid2]
  Demux1/2 -> Terminator1/1
  Theta/1 -> [Theta2]
  Iabc_out/1 -> [Iabc_out2]
  [Iabc_out2] -> I_abc_out/1
  PLL (3ph)/2 -> Terminator/1
  PLL (3ph)/1 -> Scope/1
  [Theta2] -> abc to dq0/2
  Demux2/1 -> [Idq_pcc2]
  abc to dq2/1 -> Demux2/1
  [Theta2] -> abc to dq2/2
  Demux2/2 -> Terminator2/1
  [Iabc_gc2] -> abc to dq2/1
  abc to dq3/1 -> Demux4/1
  [Theta2] -> abc to dq3/2
  Demux4/2 -> Terminator4/1
  Demux4/1 -> Vdq_pcc/1
  [Theta2] -> abc to dq4/2
  Demux5/2 -> Terminator5/1
  Demux5/1 -> Idq_pcc/1
  abc to dq4/1 -> Demux5/1
  Demux6/2 -> Terminator6/1
  abc to dq5/1 -> Demux6/1
  Demux6/1 -> Idq_inverter/1
  [Theta2] -> abc to dq5/2
  Vabc_pcc/1 -> abc to dq3/1
  Iabc_pcc/1 -> abc to dq4/1
  Iabc_inverter/1 -> abc to dq5/1

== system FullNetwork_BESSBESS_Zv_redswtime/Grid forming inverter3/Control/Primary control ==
  Vabc_pu : Inport
  Iabc_pu : Inport  Port=2
  Pref_pu : Inport  Port=3
  Qref_pu : Inport  Port=4
  Droop : Subsystem  VariantControl=ControlType == 1
  Virtual synchronous machine : Subsystem  VariantControl=ControlType == 2
  Theta : Outport
  Vd_ref : Outport  Port=2
  Vq_ref : Outport  Port=3
  w_droop : Outport  Port=4

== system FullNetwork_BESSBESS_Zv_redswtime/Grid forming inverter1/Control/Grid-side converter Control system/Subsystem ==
  Vd : Inport
  Id : Inport  Port=2
  Vd_ref : Inport  Port=3
  Itd : Inport  Port=4
  w : Inport  Port=5
  Itq : Inport  Port=6
  Vq_ref : Inport  Port=7
  Iq : Inport  Port=8
  Vq : Inport  Port=9
  Inner loops : Subsystem  VariantControl=Innerloops == 1
  No inner loops : Subsystem  VariantControl=Innerloops == 2
  Vd inverter : Outport
  Vq inverter : Outport  Port=2

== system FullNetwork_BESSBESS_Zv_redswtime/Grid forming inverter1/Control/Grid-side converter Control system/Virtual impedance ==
  Vd_ref : Inport
  Id : Inport  Port=2
  Iq : Inport  Port=3
  Vq_ref : Inport  Port=4
  No virtual impedance : Subsystem  VariantControl=Virtualimpedance == 2
  Virtual impedance : Subsystem  VariantControl=Virtualimpedance == 1
  Vd_ref* : Outport
  Vq_ref* : Outport  Port=2

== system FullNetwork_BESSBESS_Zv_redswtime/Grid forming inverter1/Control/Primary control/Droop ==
  Vabc_pu : Inport
  Iabc_pu : Inport  Port=2
  Pref_pu : Inport  Port=3
  Qref_pu : Inport  Port=4
  Constant : Constant  Value=0
  Constant1 : Constant  Value=Vnom*(sqrt(2/3))
  Constant4 : Constant  Value=2*pi
  Discrete-Time Integrator : DiscreteIntegrator  gainval=1  SampleTime=Ts  ICPrevOutput=DiscIntNeverNeededParam  ICPrevScaledInput=DiscIntNeverNeededParam
  Discrete-Time Integrator1 : DiscreteIntegrator  gainval=Ki_q  SampleTime=Ts  ICPrevOutput=DiscIntNeverNeededParam  ICPrevScaledInput=DiscIntNeverNeededParam
  First-Order Filter : spsFirstOrderFilterLib/First-Order Filter  FilterType=Lowpass  Tc=tau  Ts=Ts  Initialize=off  Vac_Init=[0, 0, 60]  Vdc_Init=0  PlotResponse=off  FreqRange="[0,  200,  1]"
  First-Order Filter1 : spsFirstOrderFilterLib/First-Order Filter  FilterType=Lowpass  Tc=0.0001  Ts=Ts  Initialize=off  Vac_Init=[0, 0, 60]  Vdc_Init=0  PlotResponse=off  FreqRange="[0,  200,  1]"
  Math Function : Math  Operator=mod  SignedPower=on
  "Power (3ph, Instantaneous)" : spsPower3phInstantaneousLib/Power (3ph, Instantaneous)
  Ramp : simulink/Sources/Ramp  slope=563.8/20  start=0  InitialOutput=0
  Saturation : Saturate  UpperLimit=563.5  LowerLimit=0
  Scope1 : Scope
  Sum1 : Sum  Inputs=|++  InputSameDT=on  SaturateOnIntegerOverflow=on
  Sum2 : Sum  Inputs=|-+  InputSameDT=on  SaturateOnIntegerOverflow=on
  Sum3 : Sum  Inputs=++|  InputSameDT=on  SaturateOnIntegerOverflow=on
  Sum4 : Sum  Inputs=|-+  InputSameDT=on  SaturateOnIntegerOverflow=on
  Sum5 : Sum  Inputs=|++  InputSameDT=on  SaturateOnIntegerOverflow=on
  Sum6 : Sum  Inputs=|++
  mp : Gain  Gain=mp
  nq : Gain  Gain=nq
  nq{1..4} (4 alike) : Gain  Gain=0
  nq5 : Gain
  wo : Constant  Value=2*pi*fnom
  Theta : Outport
  Vd_ref : Outport  Port=2
  Vq_ref : Outport  Port=3
  w_droop : Outport  Port=4
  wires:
  Constant4/1 -> Math Function/2
  Discrete-Time Integrator/1 -> Math Function/1
  wo/1 -> Sum1/2
  Sum2/1 -> mp/1
  First-Order Filter/1 -> Sum2/1
  Pref_pu/1 -> Sum2/2
  Vabc_pu/1 -> "Power (3ph, Instantaneous)"/1
  Iabc_pu/1 -> "Power (3ph, Instantaneous)"/2
  "Power (3ph, Instantaneous)"/1 -> [P_meas]
  "Power (3ph, Instantaneous)"/2 -> [Q_meas]
  [P_meas] -> First-Order Filter/1
  Constant/1 -> Vq_ref/1
  Sum6/1 -> Sum5/2, Scope1/1
  nq/1 -> Sum3/2
  Sum4/1 -> Discrete-Time Integrator1/1, nq/1
  [Q_meas] -> First-Order Filter1/1
  First-Order Filter1/1 -> Sum4/1
  Qref_pu/1 -> Sum4/2
  Sum1/1 -> w_droop/1, Discrete-Time Integrator/1
  Math Function/1 -> Theta/1
  Sum5/1 -> Vd_ref/1
  mp/1 -> nq1/1
  nq1/1 -> Sum1/1
  Sum3/1 -> nq2/1
  nq2/1 -> Sum5/1
  Discrete-Time Integrator1/1 -> nq3/1
  nq3/1 -> Sum3/1
  Ramp/1 -> Saturation/1
  Constant1/1 -> nq4/1
  Saturation/1 -> nq5/1
  nq5/1 -> Sum6/1
  nq4/1 -> Sum6/2

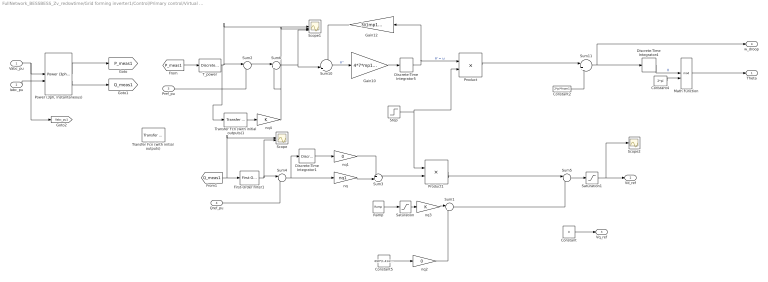
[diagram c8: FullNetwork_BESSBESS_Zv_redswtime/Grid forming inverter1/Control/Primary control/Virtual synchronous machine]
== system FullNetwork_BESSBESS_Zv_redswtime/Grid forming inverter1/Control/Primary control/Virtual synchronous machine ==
  Vabc_pu : Inport
  Iabc_pu : Inport  Port=2
  Pref_pu : Inport  Port=3
  Qref_pu : Inport  Port=4
  Constant : Constant  Value=0
  Constant2 : Constant  Value=2*pi*fnom1
  Constant4 : Constant  Value=2*pi
  Constant5 : Constant  Value=690*(1.414/1.732)
  Discrete-Time Integrator1 : DiscreteIntegrator  gainval=Ki_q  SampleTime=Ts  ICPrevOutput=DiscIntNeverNeededParam  ICPrevScaledInput=DiscIntNeverNeededParam
  Discrete-Time Integrator4 : DiscreteIntegrator  SampleTime=-1  ICPrevOutput=DiscIntNeverNeededParam  ICPrevScaledInput=DiscIntNeverNeededParam
  Discrete-Time Integrator5 : DiscreteIntegrator  SampleTime=-1  ICPrevOutput=DiscIntNeverNeededParam  ICPrevScaledInput=DiscIntNeverNeededParam
  First-Order Filter1 : spsFirstOrderFilterLib/First-Order Filter  FilterType=Lowpass  Tc=tau1  Ts=Ts  Initialize=off  Vac_Init=[0, 0, 60]  Vdc_Init=0  PlotResponse=off  FreqRange="[0,  200,  1]"
  Gain10 : Gain  Gain=4*7*mp1*2*pi*fnom/1000
  Gain12 : Gain  Gain=3/((mp1))
  Math Function : Math  Operator=mod  SignedPower=on
  "Power (3ph, Instantaneous)" : spsPower3phInstantaneousLib/Power (3ph, Instantaneous)
  Product : Product
  Product1 : Product
  Ramp : simulink/Sources/Ramp  slope=250  start=2  InitialOutput=0
  Saturation : Saturate  UpperLimit=563.5  LowerLimit=0  LinearizeAsGain=off  ZeroCross=off
  Saturation1 : Saturate  UpperLimit=563.5*1.1  LowerLimit=0  LinearizeAsGain=off  ZeroCross=off
  Scope : Scope  NumInputPorts=2
  Scope1 : Scope  NumInputPorts=3
  Scope2 : Scope
  Step : Step  Time=2  SampleTime=0
  Sum1 : Sum  Inputs=|++  InputSameDT=on  SaturateOnIntegerOverflow=on
  Sum10 : Sum  Inputs=-|+||
  Sum11 : Sum  Inputs=|++
  Sum2 : Sum  Inputs=|-+  InputSameDT=on  SaturateOnIntegerOverflow=on
  Sum3 : Sum  Inputs=++|  InputSameDT=on  SaturateOnIntegerOverflow=on
  Sum4 : Sum  Inputs=|-+  InputSameDT=on  SaturateOnIntegerOverflow=on
  Sum5 : Sum  Inputs=|++  InputSameDT=on  SaturateOnIntegerOverflow=on
  Sum6 : Sum  Inputs=|+-  InputSameDT=on  SaturateOnIntegerOverflow=on
  T_power : powerlib_extras/Discrete  Control Blocks/Discrete 1st-Order Filter  FilterType=Lowpass  Tc=tau1  Ts=Ts  Initialize=on  Vac_Init=[0 0 0]  Vdc_Init=1  PlotResponse=off  param1=[1 500 0.1]
  Transfer Fcn (with initial outputs) : simulink_extras/Additional Linear/Transfer Fcn (with initial outputs)  N=[0.15 1]  D="[0.03  1]"  Y0=0  U0=0
  Transfer Fcn (with initial outputs)1 : simulink_extras/Additional Linear/Transfer Fcn (with initial outputs)  N=[0.2 0 ]  D=[0.2 1]  Y0=0  U0=0
  nq : Gain  Gain=nq1
  nq1 : Gain  Gain=0
  nq2 : Gain  Gain=0
  nq3 : Gain
  nq4 : Gain
  Theta : Outport
  Vd_ref : Outport  Port=2
  Vq_ref : Outport  Port=3
  w_droop : Outport  Port=4
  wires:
  Constant4/1 -> Math Function/2
  T_power/1 -> Transfer Fcn (with initial outputs)1/1, Scope1/1, Sum2/1
  Pref_pu/1 -> Sum2/2
  Vabc_pu/1 -> [Vabc_pu1], "Power (3ph, Instantaneous)"/1
  Iabc_pu/1 -> "Power (3ph, Instantaneous)"/2
  "Power (3ph, Instantaneous)"/1 -> [P_meas1]
  "Power (3ph, Instantaneous)"/2 -> [Q_meas1]
  Math Function/1 -> Theta/1
  Discrete-Time Integrator5/1 -> Product/1, Gain12/1  "θ' = ω"
  Discrete-Time Integrator4/1 -> Math Function/1  "θ"
  Sum10/1 -> Gain10/1  "θ''"
  Gain10/1 -> Discrete-Time Integrator5/1
  Gain12/1 -> Sum10/1
  Sum11/1 -> Discrete-Time Integrator4/1, w_droop/1
  Constant2/1 -> Sum11/2
  nq/1 -> Sum3/2
  Sum4/1 -> nq/1, Discrete-Time Integrator1/1
  First-Order Filter1/1 -> Scope/2, Sum4/1
  [Q_meas1] -> Scope/1, First-Order Filter1/1
  Qref_pu/1 -> Sum4/2
  Constant/1 -> Vq_ref/1
  Discrete-Time Integrator1/1 -> nq1/1
  nq1/1 -> Sum3/1
  Sum3/1 -> Product1/2
  Product1/1 -> Sum5/1
  Ramp/1 -> Saturation/1
  Product/1 -> Sum11/1
  Step/1 -> Product/2, Product1/1
  Sum1/1 -> Sum5/2
  Constant5/1 -> nq2/1
  nq2/1 -> Sum1/2
  Saturation/1 -> nq3/1
  nq3/1 -> Sum1/1
  Transfer Fcn (with initial outputs)1/1 -> nq4/1
  [P_meas1] -> T_power/1
  nq4/1 -> Scope1/2, Sum6/2
  Sum6/1 -> Scope1/3, Sum10/2
  Sum2/1 -> Sum6/1
  Sum5/1 -> Saturation1/1
  Saturation1/1 -> Scope2/1, Vd_ref/1

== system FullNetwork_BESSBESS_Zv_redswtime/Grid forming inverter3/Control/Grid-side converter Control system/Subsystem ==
  Vd : Inport
  Id : Inport  Port=2
  Vd_ref : Inport  Port=3
  Itd : Inport  Port=4
  w : Inport  Port=5
  Itq : Inport  Port=6
  Vq_ref : Inport  Port=7
  Iq : Inport  Port=8
  Vq : Inport  Port=9
  Inner loops : Subsystem  VariantControl=Innerloops == 1
  No inner loops : Subsystem  VariantControl=Innerloops == 2
  Vd inverter : Outport
  Vq inverter : Outport  Port=2

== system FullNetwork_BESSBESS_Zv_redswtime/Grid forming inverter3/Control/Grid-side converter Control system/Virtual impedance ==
  Vd_ref : Inport
  Id : Inport  Port=2
  Iq : Inport  Port=3
  Vq_ref : Inport  Port=4
  No virtual impedance : Subsystem  VariantControl=Virtualimpedance == 2
  Virtual impedance : Subsystem  VariantControl=Virtualimpedance == 1
  Vd_ref* : Outport
  Vq_ref* : Outport  Port=2

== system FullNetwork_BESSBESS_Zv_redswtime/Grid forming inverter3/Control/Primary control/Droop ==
  Vabc_pu : Inport
  Iabc_pu : Inport  Port=2
  Pref_pu : Inport  Port=3
  Qref_pu : Inport  Port=4
  Constant : Constant  Value=0
  Constant1 : Constant  Value=Vnom*(sqrt(2/3))
  Constant4 : Constant  Value=2*pi
  Discrete-Time Integrator : DiscreteIntegrator  gainval=1  SampleTime=Ts  ICPrevOutput=DiscIntNeverNeededParam  ICPrevScaledInput=DiscIntNeverNeededParam
  Discrete-Time Integrator1 : DiscreteIntegrator  gainval=Ki_q  SampleTime=Ts  ICPrevOutput=DiscIntNeverNeededParam  ICPrevScaledInput=DiscIntNeverNeededParam
  First-Order Filter : spsFirstOrderFilterLib/First-Order Filter  FilterType=Lowpass  Tc=tau  Ts=Ts  Initialize=off  Vac_Init=[0, 0, 60]  Vdc_Init=0  PlotResponse=off  FreqRange="[0,  200,  1]"
  First-Order Filter1 : spsFirstOrderFilterLib/First-Order Filter  FilterType=Lowpass  Tc=0.0001  Ts=Ts  Initialize=off  Vac_Init=[0, 0, 60]  Vdc_Init=0  PlotResponse=off  FreqRange="[0,  200,  1]"
  Math Function : Math  Operator=mod  SignedPower=on
  "Power (3ph, Instantaneous)" : spsPower3phInstantaneousLib/Power (3ph, Instantaneous)
  Ramp : simulink/Sources/Ramp  slope=563.8/20  start=0  InitialOutput=0
  Saturation : Saturate  UpperLimit=563.5  LowerLimit=0
  Scope1 : Scope
  Sum1 : Sum  Inputs=|++  InputSameDT=on  SaturateOnIntegerOverflow=on
  Sum2 : Sum  Inputs=|-+  InputSameDT=on  SaturateOnIntegerOverflow=on
  Sum3 : Sum  Inputs=++|  InputSameDT=on  SaturateOnIntegerOverflow=on
  Sum4 : Sum  Inputs=|-+  InputSameDT=on  SaturateOnIntegerOverflow=on
  Sum5 : Sum  Inputs=|++  InputSameDT=on  SaturateOnIntegerOverflow=on
  Sum6 : Sum  Inputs=|++
  mp : Gain  Gain=mp
  nq : Gain  Gain=nq
  nq{1..4} (4 alike) : Gain  Gain=0
  nq5 : Gain
  wo : Constant  Value=2*pi*fnom
  Theta : Outport
  Vd_ref : Outport  Port=2
  Vq_ref : Outport  Port=3
  w_droop : Outport  Port=4
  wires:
  Constant4/1 -> Math Function/2
  Discrete-Time Integrator/1 -> Math Function/1
  wo/1 -> Sum1/2
  Sum2/1 -> mp/1
  First-Order Filter/1 -> Sum2/1
  Pref_pu/1 -> Sum2/2
  Vabc_pu/1 -> "Power (3ph, Instantaneous)"/1
  Iabc_pu/1 -> "Power (3ph, Instantaneous)"/2
  "Power (3ph, Instantaneous)"/1 -> [P_meas]
  "Power (3ph, Instantaneous)"/2 -> [Q_meas]
  [P_meas] -> First-Order Filter/1
  Constant/1 -> Vq_ref/1
  Sum6/1 -> Sum5/2, Scope1/1
  nq/1 -> Sum3/2
  Sum4/1 -> Discrete-Time Integrator1/1, nq/1
  [Q_meas] -> First-Order Filter1/1
  First-Order Filter1/1 -> Sum4/1
  Qref_pu/1 -> Sum4/2
  Sum1/1 -> w_droop/1, Discrete-Time Integrator/1
  Math Function/1 -> Theta/1
  Sum5/1 -> Vd_ref/1
  mp/1 -> nq1/1
  nq1/1 -> Sum1/1
  Sum3/1 -> nq2/1
  nq2/1 -> Sum5/1
  Discrete-Time Integrator1/1 -> nq3/1
  nq3/1 -> Sum3/1
  Ramp/1 -> Saturation/1
  Constant1/1 -> nq4/1
  Saturation/1 -> nq5/1
  nq5/1 -> Sum6/1
  nq4/1 -> Sum6/2

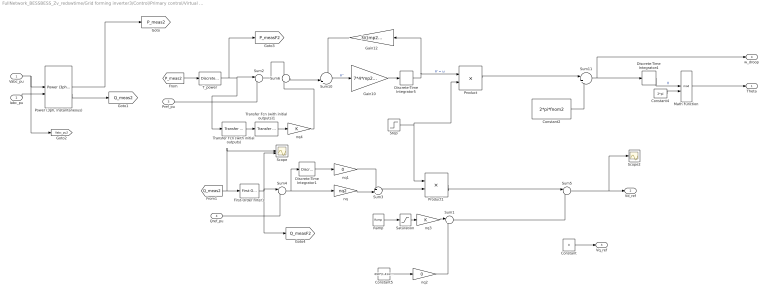
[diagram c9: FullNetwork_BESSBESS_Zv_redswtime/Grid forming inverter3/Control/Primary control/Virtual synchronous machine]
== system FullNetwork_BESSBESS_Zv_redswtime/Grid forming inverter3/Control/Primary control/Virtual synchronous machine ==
  Vabc_pu : Inport
  Iabc_pu : Inport  Port=2
  Pref_pu : Inport  Port=3
  Qref_pu : Inport  Port=4
  Constant : Constant  Value=0
  Constant2 : Constant  Value=2*pi*fnom2
  Constant4 : Constant  Value=2*pi
  Constant5 : Constant  Value=690*(1.414/1.732)
  Discrete-Time Integrator1 : DiscreteIntegrator  gainval=Ki_q  SampleTime=Ts  LimitOutput=on  ICPrevOutput=DiscIntNeverNeededParam  ICPrevScaledInput=DiscIntNeverNeededParam
  Discrete-Time Integrator4 : DiscreteIntegrator  SampleTime=-1  ICPrevOutput=DiscIntNeverNeededParam  ICPrevScaledInput=DiscIntNeverNeededParam
  Discrete-Time Integrator5 : DiscreteIntegrator  SampleTime=-1  ICPrevOutput=DiscIntNeverNeededParam  ICPrevScaledInput=DiscIntNeverNeededParam
  First-Order Filter1 : spsFirstOrderFilterLib/First-Order Filter  FilterType=Lowpass  Tc=tau2  Ts=Ts  Initialize=off  Vac_Init=[0, 0, 60]  Vdc_Init=0  PlotResponse=off  FreqRange="[0,  200,  1]"
  Gain10 : Gain  Gain=7*4*mp2*2*pi*fnom/1000
  Gain12 : Gain  Gain=3/((mp2))
  Math Function : Math  Operator=mod  SignedPower=on
  "Power (3ph, Instantaneous)" : spsPower3phInstantaneousLib/Power (3ph, Instantaneous)
  Product : Product
  Product1 : Product
  Ramp : simulink/Sources/Ramp  slope=250  start=2  InitialOutput=0
  Saturation : Saturate  UpperLimit=563.5  LowerLimit=0  LinearizeAsGain=off  ZeroCross=off
  Scope : Scope  NumInputPorts=2
  Scope2 : Scope
  Step : Step  Time=0  SampleTime=0
  Sum1 : Sum  Inputs=|++  InputSameDT=on  SaturateOnIntegerOverflow=on
  Sum10 : Sum  Inputs=-|+||
  Sum11 : Sum  Inputs=|++
  Sum2 : Sum  Inputs=|-+  InputSameDT=on  SaturateOnIntegerOverflow=on
  Sum3 : Sum  Inputs=++|  InputSameDT=on  SaturateOnIntegerOverflow=on
  Sum4 : Sum  Inputs=|-+  InputSameDT=on  SaturateOnIntegerOverflow=on
  Sum5 : Sum  Inputs=|++  InputSameDT=on  SaturateOnIntegerOverflow=on
  Sum6 : Sum  Inputs=+-  InputSameDT=on  SaturateOnIntegerOverflow=on
  T_power : powerlib_extras/Discrete  Control Blocks/Discrete 1st-Order Filter  FilterType=Lowpass  Tc=tau2  Ts=Ts  Initialize=on  Vac_Init=[0 0 0]  Vdc_Init=1  PlotResponse=off  param1=[1 500 0.1]
  Transfer Fcn (with initial outputs) : simulink_extras/Additional Linear/Transfer Fcn (with initial outputs)  N=[0.15 1]  D="[0.03  1]"  Y0=0  U0=0
  Transfer Fcn (with initial outputs)1 : simulink_extras/Additional Linear/Transfer Fcn (with initial outputs)  N=[0.2 0 ]  D=[0.2 1]  Y0=0  U0=0
  nq : Gain  Gain=nq2
  nq1 : Gain  Gain=0
  nq2 : Gain  Gain=0
  nq3 : Gain
  nq4 : Gain
  Theta : Outport
  Vd_ref : Outport  Port=2
  Vq_ref : Outport  Port=3
  w_droop : Outport  Port=4
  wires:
  Constant4/1 -> Math Function/2
  Pref_pu/1 -> Sum2/2
  Vabc_pu/1 -> [Vabc_pu2], "Power (3ph, Instantaneous)"/1
  Iabc_pu/1 -> "Power (3ph, Instantaneous)"/2
  "Power (3ph, Instantaneous)"/1 -> [P_meas2]
  "Power (3ph, Instantaneous)"/2 -> [Q_meas2]
  [P_meas2] -> T_power/1
  Math Function/1 -> Theta/1
  Discrete-Time Integrator5/1 -> Product/1, Gain12/1  "θ' = ω"
  Discrete-Time Integrator4/1 -> Math Function/1  "θ"
  Sum10/1 -> Gain10/1  "θ''"
  Gain10/1 -> Discrete-Time Integrator5/1
  Gain12/1 -> Sum10/1
  Sum11/1 -> Discrete-Time Integrator4/1, w_droop/1
  Constant2/1 -> Sum11/2
  nq/1 -> Sum3/2
  Sum4/1 -> nq/1, Discrete-Time Integrator1/1
  First-Order Filter1/1 -> [Q_measF2], Scope/2, Sum4/1
  [Q_meas2] -> Scope/1, First-Order Filter1/1
  Qref_pu/1 -> Sum4/2
  Constant/1 -> Vq_ref/1
  Discrete-Time Integrator1/1 -> nq1/1
  nq1/1 -> Sum3/1
  Sum3/1 -> Product1/2
  Product1/1 -> Sum5/1
  Ramp/1 -> Saturation/1
  Product/1 -> Sum11/1
  Step/1 -> Product/2, Product1/1
  Sum1/1 -> Sum5/2
  Constant5/1 -> nq2/1
  nq2/1 -> Sum1/2
  Saturation/1 -> nq3/1
  nq3/1 -> Sum1/1
  Sum5/1 -> Scope2/1, Vd_ref/1
  Transfer Fcn (with initial outputs)/1 -> Transfer Fcn (with initial outputs)1/1
  Transfer Fcn (with initial outputs)1/1 -> nq4/1
  T_power/1 -> [P_measF2], Transfer Fcn (with initial outputs)/1, Sum2/1
  Sum2/1 -> Sum6/1
  Sum6/1 -> Sum10/2
  nq4/1 -> Sum6/2
